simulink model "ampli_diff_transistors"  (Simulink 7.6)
settings: Solver=ode15s  StartTime=0.0  StopTime=.2  RelTol=1e-3
StopFcn:
  | close all, clc
  | load  ES_ampli_diff.mat
  | plotyy(x(1,:),x(2,:),x(1,:),x(3,:))
  | grid
  | title('Tension de sortie et courant de collecteur - Ampli différentiel')
  | xlabel('temps')
libraries: fl_lib x13, elec_lib x3, nesl_utility x3

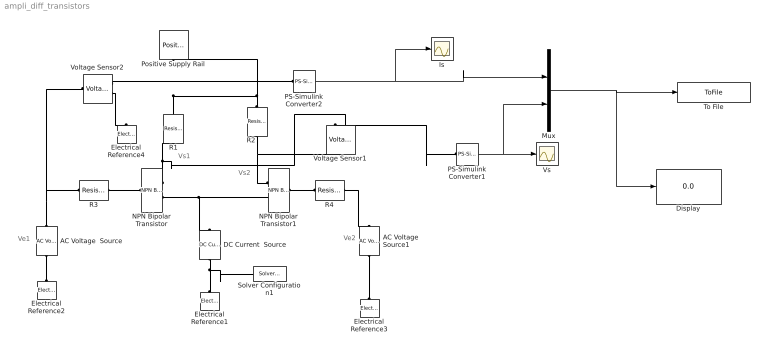
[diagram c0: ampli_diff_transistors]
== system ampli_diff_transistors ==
  note: Ve1
  note: Ve2
  note: Vs1
  note: Vs2
  AC Voltage  Source : fl_lib/Electrical/Electrical Sources/AC Voltage Source  DialogController=NetworkEngine.DynNeDlgSource  SystemSampleTime=-1  amp=1.1 V  shift=0 rad  omega=10 Hz  i_Log=off  v_Log=off  LocalVarNames=|current|voltage|power  LocalVarDescs=|Current (A)|Voltage (V)|Power (W)  LocalVarLogging=[0 0 0]
  AC Voltage  Source1 : fl_lib/Electrical/Electrical Sources/AC Voltage Source  DialogController=NetworkEngine.DynNeDlgSource  SystemSampleTime=-1  amp=1 V  shift=0 rad  omega=10 Hz  i_Log=off  v_Log=off  LocalVarNames=|current|voltage|power  LocalVarDescs=|Current (A)|Voltage (V)|Power (W)  LocalVarLogging=[0 0 0]
  DC Current  Source : fl_lib/Electrical/Electrical Sources/DC Current Source  DialogController=NetworkEngine.DynNeDlgSource  SystemSampleTime=-1  i0=3 mA  i_Log=off  v_Log=off  LocalVarNames=|i|v  LocalVarDescs=|i|v  LocalVarLogging=[0 0]
  Display : Display
  Electrical Reference{1..4} (4 alike) : fl_lib/Electrical/Electrical Elements/Electrical Reference  DialogController=NetworkEngine.DynNeDlgSource  SystemSampleTime=-1  i_Log=off  LocalVarNames=|i  LocalVarDescs=|i  LocalVarLogging=[]
  Is : Scope
  Mux : Mux  Inputs=2
  NPN Bipolar Transistor : elec_lib/Semiconductor Devices/NPN Bipolar Transistor  DialogController=NetworkEngine.DynNeDlgSource  SystemSampleTime=-1  parameterization=1  BF=100  IS=1e-14 A  VAF=200 V  hfe=100  hoe=5e-5 1/Ohm  Ic_h=1 mA  V1=0.55 V  I1=0.5 mA  BR=1  Tmeas=25 C  RC=0.01 Ohm  RE=1e-4 Ohm  RB=1 Ohm  C_BC=5 pF  C_BE=5 pF  TF=0 us  TR=0 us  LocalVarLogging=[]
  NPN Bipolar Transistor1 : elec_lib/Semiconductor Devices/NPN Bipolar Transistor  DialogController=NetworkEngine.DynNeDlgSource  SystemSampleTime=-1  parameterization=1  BF=100  IS=1e-14 A  VAF=200 V  hfe=100  hoe=5e-5 1/Ohm  Ic_h=1 mA  V1=0.55 V  I1=0.5 mA  BR=1  Tmeas=25 C  RC=0.01 Ohm  RE=1e-4 Ohm  RB=1 Ohm  C_BC=5 pF  C_BE=5 pF  TF=0 us  TR=0 us  LocalVarLogging=[]
  PS-Simulink Converter1 : nesl_utility/PS-Simulink Converter  DialogController=NetworkEngine.DynNeUtilDlgSource  SystemSampleTime=-1  PhysicalDomain=network_engine_domain  LeftPortType=input  RightPortType=output  SubClassName=ps_output  Unit=1  AffineConversion=off
  PS-Simulink Converter2 : nesl_utility/PS-Simulink Converter  DialogController=NetworkEngine.DynNeUtilDlgSource  SystemSampleTime=-1  PhysicalDomain=network_engine_domain  LeftPortType=input  RightPortType=output  SubClassName=ps_output  Unit=1  AffineConversion=off
  Positive Supply Rail : elec_lib/Sources/Positive Supply Rail  DialogController=NetworkEngine.DynNeDlgSource  SystemSampleTime=-1  v0=12 V  current_Log=off  voltage_Log=off  power_Log=off  LocalVarNames=|current|voltage|power  LocalVarDescs=|Current (A)|Voltage (V)|Power (W)  LocalVarLogging=[0 0 0]
  R1 : fl_lib/Electrical/Electrical Elements/Resistor  DialogController=NetworkEngine.DynNeDlgSource  SystemSampleTime=-1  R=4.7 kOhm  i_Log=off  v_Log=off  LocalVarNames=|current|voltage|power  LocalVarDescs=|Resistor current (A)|Voltage across resistor (V)|Power (W)  LocalVarLogging=[0 0 0]
  R2 : fl_lib/Electrical/Electrical Elements/Resistor  DialogController=NetworkEngine.DynNeDlgSource  SystemSampleTime=-1  R=4.7 kOhm  i_Log=off  v_Log=off  LocalVarNames=|current|voltage|power  LocalVarDescs=|Resistor current (A)|Voltage across resistor (V)|Power (W)  LocalVarLogging=[0 0 0]
  R3 : fl_lib/Electrical/Electrical Elements/Resistor  DialogController=NetworkEngine.DynNeDlgSource  SystemSampleTime=-1  R=10 kOhm  i_Log=off  v_Log=off  LocalVarNames=|current|voltage|power  LocalVarDescs=|Resistor current (A)|Voltage across resistor (V)|Power (W)  LocalVarLogging=[0 0 0]
  R4 : fl_lib/Electrical/Electrical Elements/Resistor  DialogController=NetworkEngine.DynNeDlgSource  SystemSampleTime=-1  R=10 kOhm  i_Log=off  v_Log=off  LocalVarNames=|current|voltage|power  LocalVarDescs=|Resistor current (A)|Voltage across resistor (V)|Power (W)  LocalVarLogging=[0 0 0]
  Solver Configuration1 : nesl_utility/Solver Configuration  DialogController=NetworkEngine.DynNeUtilDlgSource  SystemSampleTime=-1  PhysicalDomain=network_engine_domain  LeftPortType=input  RightPortType=generic  SubClassName=solver  Accelerate=off  Profile=off  ResidualTolerance=1e-9  MaxNonlinIter=12  MaxModeIter=2  DoFixedCost=off  UseLocalSampling=off  DoDC=off  LinearAlgebra=Sparse  LocalSolverSampleTime=.001  LocalSolverChoice=NE_BACKWARD_EULER_ADVANCER  UseLocalSolver=off
  To File : ToFile  Filename=ES_ampli_diff  MatrixName=x
  Voltage Sensor1 : fl_lib/Electrical/Electrical Sensors/Voltage Sensor  DialogController=NetworkEngine.DynNeDlgSource  SystemSampleTime=-1  i1_Log=off  v1_Log=off  LocalVarNames=|i1|v1  LocalVarDescs=|i1|v1  LocalVarLogging=[]
  Voltage Sensor2 : fl_lib/Electrical/Electrical Sensors/Voltage Sensor  DialogController=NetworkEngine.DynNeDlgSource  SystemSampleTime=-1  i1_Log=off  v1_Log=off  LocalVarNames=|i1|v1  LocalVarDescs=|i1|v1  LocalVarLogging=[]
  Vs : Scope
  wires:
  Mux/1 -> To File/1, Display/1
  PS-Simulink Converter2/1 -> Mux/1, Is/1
  PS-Simulink Converter1/1 -> Mux/2, Vs/1
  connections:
  DC Current  Source/LConn1 -- Electrical Reference1/LConn1 -- Solver Configuration1/RConn1
  NPN Bipolar Transistor/RConn2 -- DC Current  Source/RConn1 -- NPN Bipolar Transistor1/RConn2
  NPN Bipolar Transistor/RConn1 -- R1/RConn1 -- Voltage Sensor1/RConn2
  R2/RConn1 -- NPN Bipolar Transistor1/RConn1 -- Voltage Sensor1/LConn1
  AC Voltage  Source/LConn1 -- R3/LConn1 -- Voltage Sensor2/LConn1
  R3/RConn1 -- NPN Bipolar Transistor/LConn1
  AC Voltage  Source/RConn1 -- Electrical Reference2/LConn1
  Electrical Reference3/LConn1 -- AC Voltage  Source1/RConn1
  R4/RConn1 -- AC Voltage  Source1/LConn1
  NPN Bipolar Transistor1/LConn1 -- R4/LConn1
  R2/LConn1 -- R1/LConn1 -- Positive Supply Rail/RConn1
  Voltage Sensor1/RConn1 -- PS-Simulink Converter1/LConn1
  Voltage Sensor2/RConn2 -- Electrical Reference4/LConn1
  Voltage Sensor2/RConn1 -- PS-Simulink Converter2/LConn1
